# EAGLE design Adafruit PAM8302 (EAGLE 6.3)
COMPANY: ADAFRUIT INDUSTRIES; DRAWN: KTOWN; REV: A
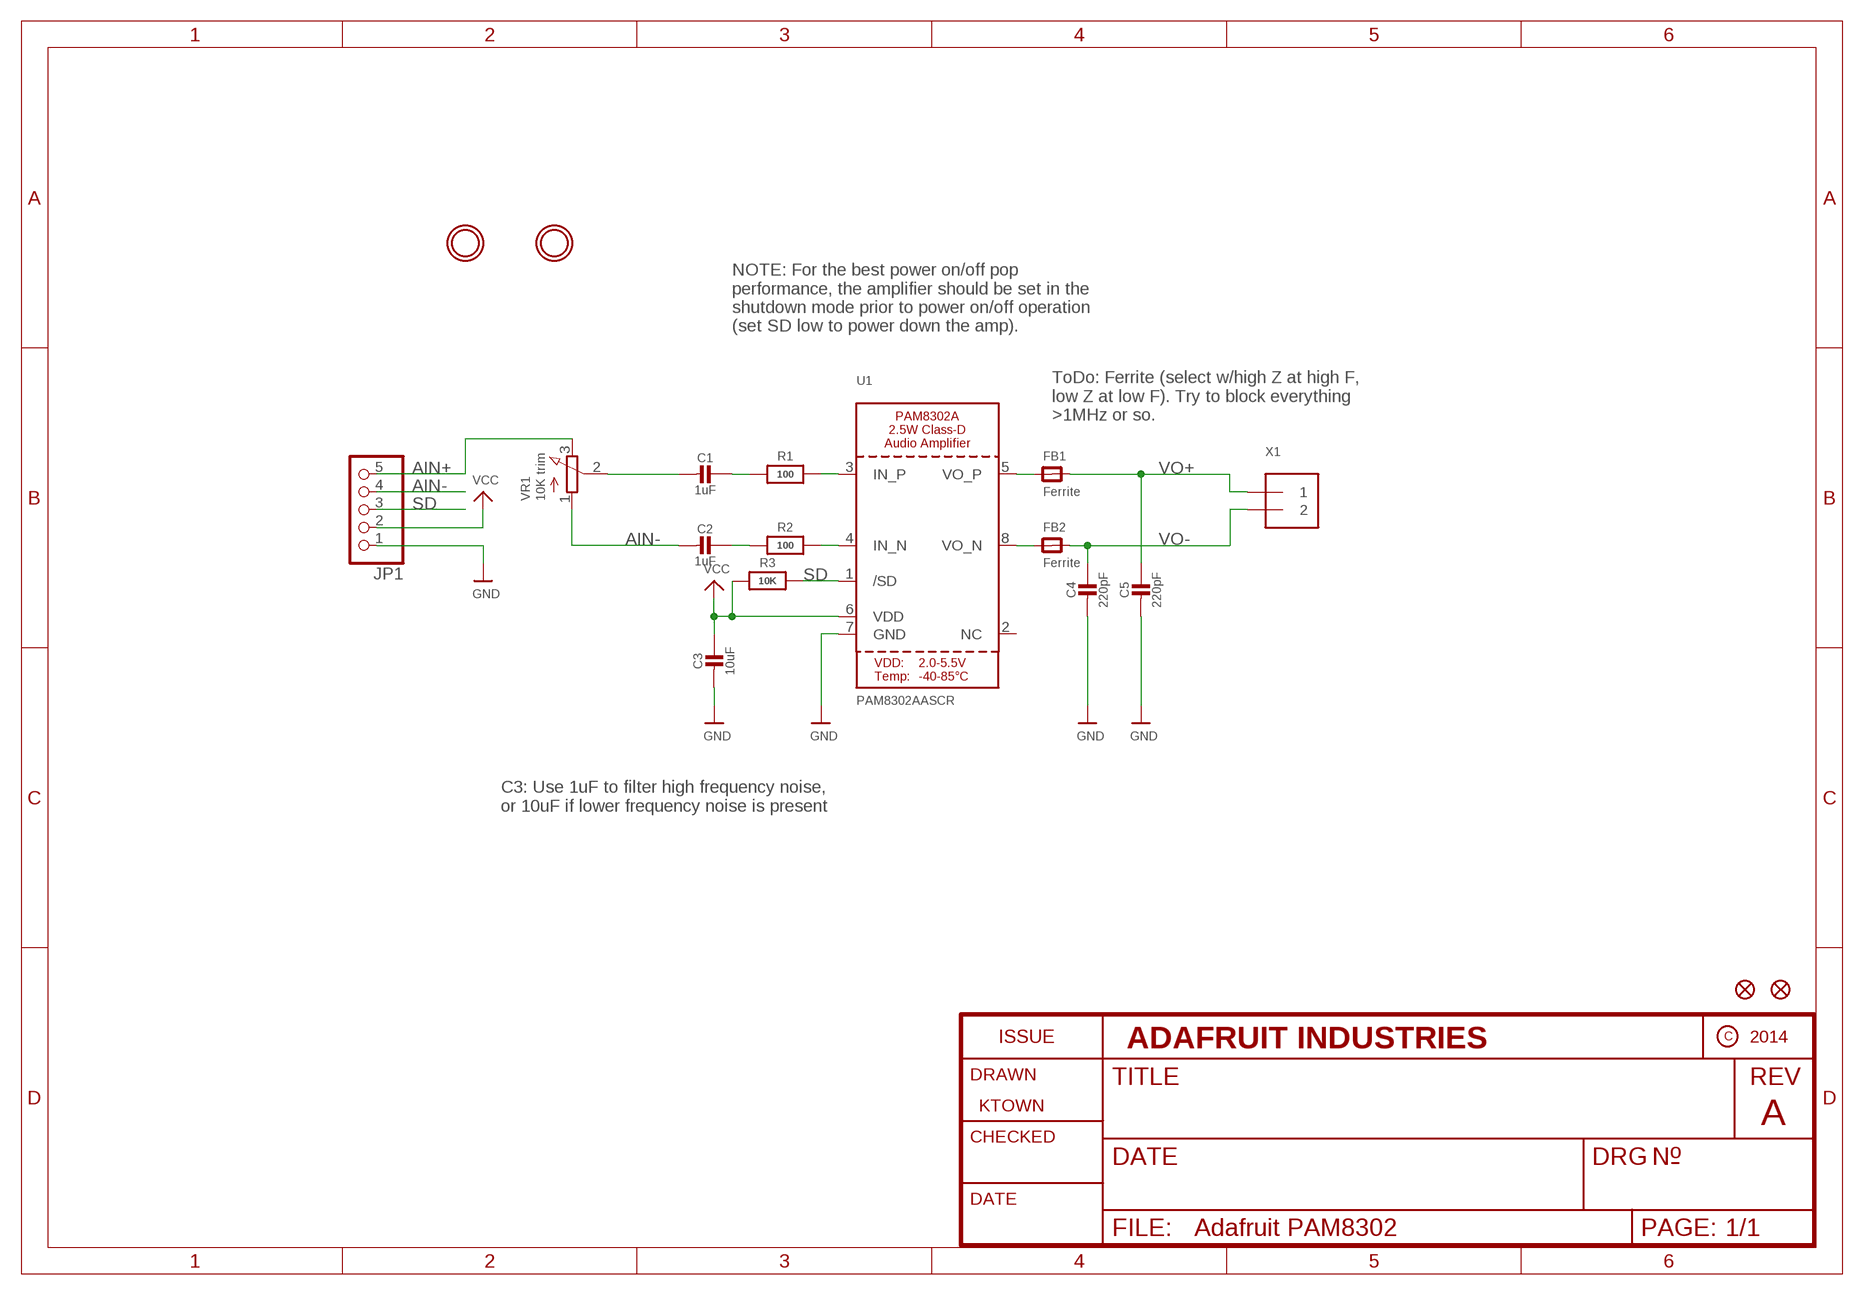
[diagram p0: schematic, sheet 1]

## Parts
C1  1uF  CAP_CERAMIC0805-NOOUTLINE  [0805-NO]
C2  1uF  CAP_CERAMIC0805-NOOUTLINE  [0805-NO]
C3  10uF  CAP_CERAMIC0805-NOOUTLINE  [0805-NO]
C4  220pF  CAP_CERAMIC0805-NOOUTLINE  [0805-NO]
C5  220pF  CAP_CERAMIC0805-NOOUTLINE  [0805-NO]
FB1  Ferrite  FERRITE_0805  [_0805]
FB2  Ferrite  FERRITE_0805  [_0805]
FID1  FIDUCIAL""  [FIDUCIAL_1MM]
FID2  FIDUCIAL""  [FIDUCIAL_1MM]
JP1  HEADER-1X570MIL  [1X05_ROUND_70]
R1  100  RESISTOR0805_NOOUTLINE  [0805-NO]
R2  100  RESISTOR0805_NOOUTLINE  [0805-NO]
R3  10K  RESISTOR0805_NOOUTLINE  [0805-NO]
U1  PAM8302AASCR  AUDIOAMP_PAM8302A  [MSOP8_0.65MM]
U$10  MOUNTINGHOLE2.0  [MOUNTINGHOLE_2.0_PLATED]
U$11  MOUNTINGHOLE2.0  [MOUNTINGHOLE_2.0_PLATED]
VR1  10K trim  TRIMPOT3303W/X  [TRIMPOT_BOURNS_3303W]
X1  TERMBLOCK_1X2  [TERMBLOCK_1X2-3.5MM]

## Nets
AIN+: JP1.5 VR1.3(E)
AIN-: C2.2 JP1.4 VR1.1(A)
GND: C3.2 C4.2 C5.2 JP1.1 U1.7(GND)
N$1: R2.2 U1.4(IN_N)
N$2: R1.2 U1.3(IN_P)
N$3: C1.1 R1.1
N$4: C2.1 R2.1
N$5: FB2.1 U1.8(VO_N)
N$6: FB1.1 U1.5(VO_P)
N$7: C1.2 VR1.2(S)
SD: JP1.3 R3.2 U1.1(/SD)
VCC: C3.1 JP1.2 R3.1 U1.6(VDD)
VO+: C5.1 FB1.2 X1.1
VO-: C4.1 FB2.2 X1.2
Unconnected: U1.2(NC)

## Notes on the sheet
- NOTE: For the best power on/off pop
  performance, the amplifier should be set in the
  shutdown mode prior to power on/off operation
  (set SD low to power down the amp).
- ToDo: Ferrite (select w/high Z at high F,
  low Z at low F). Try to block everything
  >1MHz or so.
- C3: Use 1uF to filter high frequency noise,
  or 10uF if lower frequency noise is present

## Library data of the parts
C1-C5 = microbuilder:CAP_CERAMIC: Ceramic Capacitors
FB1 FB2 = microbuilder:FERRITE: Ferrite Bead
FID1 FID2 = microbuilder:FIDUCIAL: Fiducial Alignment Points; BOM: EXCLUDE
JP1 = microbuilder:HEADER-1X5: PIN HEADER
R1-R3 = microbuilder:RESISTOR: Resistors
U1 = microbuilder:AUDIOAMP_PAM8302A: PAM8302A - 2.5W Class-D Mono Audio Amplifier MSOP8 = PAM8302AASCR
U$10 U$11 = microbuilder:MOUNTINGHOLE: Mounting Hole; BOM: EXCLUDE
VR1 = microbuilder:TRIMPOT: 3-Pin SMT Trimpots Bourns TC33 (X-2) Series 1K - Digikey: TC33X-102ECT-ND 10K - Digikey: TC33X-2-103E 100K - Digikey: TC33X-104ECT-ND Bourns 3303 (W) Series 3mm 10K Single Turn - Digikey: 3303W-103ETR-ND 3mm 100K Single Turn - Digikey: 3303X-104ETR-ND
X1 = microbuilder:TERMBLOCK_1X2: 3.5mm Terminal block

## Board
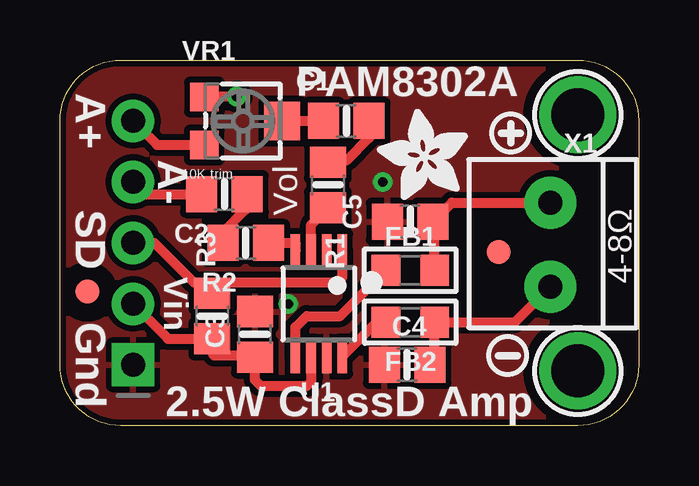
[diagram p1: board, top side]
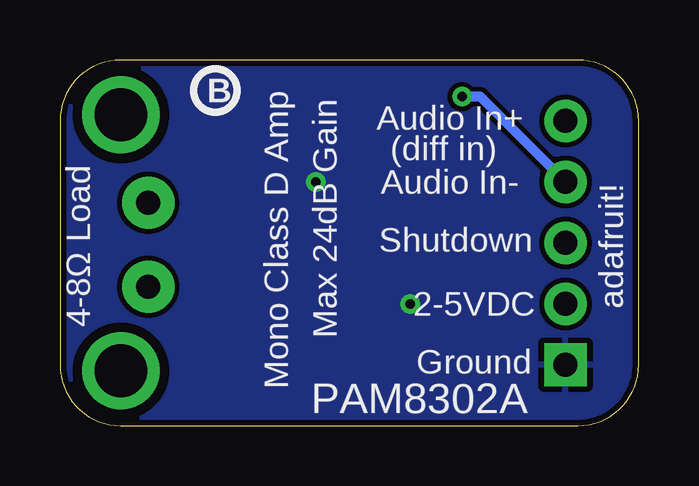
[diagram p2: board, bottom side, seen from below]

Size 24.13 x 15.24 mm. Coordinates in mm from the lower left corner, seen from the top.
Outline: 0,2.54 0,12.7 arc-90 2.54,15.24 21.59,15.24 arc-90 24.13,12.7 24.13,2.54 arc-90 21.59,0 2.54,0 arc-90 0,2.54
Copper layers (1*16): Top 0.035mm / dielectric 1.5mm / Bottom 0.035mm
Design rules "adafruit": minimum track width 8mil, minimum drill 15.5mil, track to track 8mil, track to pad 8mil, pad to pad 8mil, via to via 8mil, smd to smd 8mil, copper to edge 10mil, drill to drill 8mil, minimum pad ring 10mil, minimum via ring 8mil, stop-mask expansion 2mil, vias tented up to drill 20mil, thermal gap 10mil

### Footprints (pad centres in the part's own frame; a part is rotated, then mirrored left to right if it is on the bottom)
0805-NO = smd 1.3 x 1.5: 1 -0.95,0; 2 0.95,0
_0805 = smd 1.2 x 1.3: 1 -1.016,0; 2 1.016,0
FIDUCIAL_1MM = smd 1 x 1: 1 0,0
1X05_ROUND_70 = drill 1 pad 1.778 square: 1 -5.08,0 | drill 1 pad 1.778: 2 -2.54,0; 3 0,0; 4 2.54,0; 5 5.08,0
MSOP8_0.65MM = smd 0.4 x 1.4: 1 -0.975,-2.2; 2 -0.325,-2.2; 3 0.325,-2.2; 4 0.975,-2.2; 5 0.975,2.2; 6 0.325,2.2; 7 -0.325,2.2; 8 -0.975,2.2
MOUNTINGHOLE_2.0_PLATED = drill 2.2 pad 3: P$1 0,0
TRIMPOT_BOURNS_3303W = smd 1.2 x 1.2: 1 -1,-1.6; 3 1,-1.6 | smd 1.6 x 1.5: 2 0,1.65
TERMBLOCK_1X2-3.5MM = drill 1 pad 2.184: 1 1.8,0; 2 -1.7,0

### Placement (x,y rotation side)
C1  11.94,12.7 180 top
C2  6.86,9.65 180 top
C3  8.13,3.81 90 top
C4  14.48,2.54 180 top
C5  14.61,8.51 180 top
FB1  14.61,6.48 0 top
FB2  14.61,4.32 0 top
FID1  18.29,7.24 0 top
FID2  1.14,5.59 0 top
JP1  3.05,7.62 90 top
R1  11.18,10.03 270 top
R2  7.75,7.62 0 top
R3  6.35,4.57 90 top
U1  10.79,5.08 180 top
U$3  [SYMBOL_PLUS]  18.8,12.19 180 top
U$4  [SYMBOL_MINUS]  18.67,2.92 0 top
U$5  [ADAFRUIT_3.5MM]  17.02,9.4 90 top
U$6  [PCBFEAT-REV-040]  17.65,13.97 0 bottom
U$10  21.59,12.95 0 top
U$11  21.59,2.29 0 top
VR1  7.62,12.7 270 top
X1  20.45,7.49 90 top

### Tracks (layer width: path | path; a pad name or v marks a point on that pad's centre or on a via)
AIN+
  Top 0.406: JP1.5 4.05,11.7 VR1.3
AIN-  (via drill 0.4)
  Top 0.406: JP1.4 3.56,9.65 C2.2 | v7.37,13.72 7.48,13.7 VR1.1
  Bottom 0.406: JP1.4 6.6,13.72 v7.37,13.72
GND  (via drill 0.4)
  other vias: 13.46,10.16 9.53,5.08
  pour Top (isolate 0.254): 0,2.54 0,12.7 arc-90 2.54,15.24 21.59,15.24 arc-90 24.13,12.7 24.13,2.54 arc-90 21.59,0 2.54,0 arc-90
  pour Bottom: -0.38,15.37 -0.38,-0.13 24.26,-0.13 24.26,15.37
N$1
  Top 0.406: R2.2 9.82,7.62 U1.4
N$2
  Top 0.406: U1.3 10.47,8.38 R1.2
N$3
  Top 0.406: C1.1 12.89,12 11.94,11.05 11.24,11.05 R1.1
N$4
  Top 0.406: R2.1 6.8,8.07 7.75,9.02 7.75,9.59 C2.1
N$5
  Top 0.406: U1.8 13.21,4.32 FB2.1
N$6
  Top 0.406: U1.5 9.82,4.11 10.29,4.57 11.68,4.57 FB1.1 13.08,5.84
N$7
  Top 0.406: VR1.2 C1.2
SD
  Top 0.406: U1.1 11.77,6.18 11.56,5.97 6.35,5.97 | 6.35,5.97 5.59,5.97 3.94,7.62 JP1.3 | R3.2 6.35,5.97
VCC
  Top 0.406: U1.6 10.47,1.83 10.29,1.65 8.38,1.65 8.13,1.91 C3.1 7.94,2.92 6.41,2.92 R3.1 4.51,3.62 JP1.2
VO+
  Top 0.406: FB1.2 15.62,8.44 C5.1 16.34,9.29 X1.1
VO-
  Top 0.406: C4.1 15.62,2.73 FB2.2 18.97,4.32 X1.2

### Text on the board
tPlace: PAM8302A | A+ | A- | Vol | SD | 4-8Ω | Vin | Gnd | 2.5W ClassD Amp
bPlace: Audio In+ | (diff in) | Audio In- | Max 24dB Gain | Shutdown | Mono Class D Amp | adafruit! | 4-8Ω Load | 2-5VDC | Ground | PAM8302A

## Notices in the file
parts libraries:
microbuilder: This work is placed in the public domain, and may be freely used for commercial and non-commercial work with the following conditions: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
